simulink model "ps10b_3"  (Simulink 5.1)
settings: Solver=ode45  StartTime=0.0  StopTime=10.0  RelTol=1e-3
undefined symbols (not defined in the file or in its folder): Ak, Bk, Ck, Dk

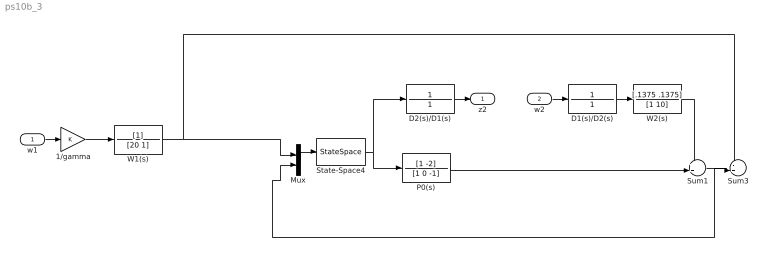
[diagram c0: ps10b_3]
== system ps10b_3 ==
  w1 : Inport
  w2 : Inport  Port=2
  1/gamma : Gain
  D1(s)/D2(s) : TransferFcn  Numerator=1  Denominator=1
  D2(s)/D1(s) : TransferFcn  Numerator=1  Denominator=1
  Mux : Mux  Inputs=2
  P0(s) : TransferFcn  Numerator=[1 -2]  Denominator=[1 0 -1]
  State-Space4 : StateSpace  A=Ak  B=Bk  C=Ck  D=Dk
  Sum1 : Sum  Inputs=++|
  Sum3 : Sum  Inputs=-+|
  W1(s) : TransferFcn  Denominator=[20 1]
  W2(s) : TransferFcn  Numerator=[.1375 .1375]  Denominator=[1 10]
  z2 : Outport
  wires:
  1/gamma/1 -> W1(s)/1
  W1(s)/1 -> Sum3/1, Mux/1
  D2(s)/D1(s)/1 -> z2/1
  w2/1 -> D1(s)/D2(s)/1
  D1(s)/D2(s)/1 -> W2(s)/1
  W2(s)/1 -> Sum1/1
  P0(s)/1 -> Sum1/2
  Sum1/1 -> Sum3/2, Mux/2
  Sum3/1 -> ?
  Mux/1 -> State-Space4/1
  State-Space4/1 -> P0(s)/1, D2(s)/D1(s)/1
  w1/1 -> 1/gamma/1
